(* Logix 5000 AddOnInstructionDefinition export Banner_B25_PD_v4; software revision 33.03 *)

TYPE Banner_B25_PDI_v4 :   // Process Data for a B25. This will include event information.
STRUCT
   Output_State : SINT;   // 0 = Inactive, 1 = Active
   Marginal_Signal : SINT;   // 0 = Normal, 1 = Marginal
END_STRUCT
END_TYPE

ADD_ON_INSTRUCTION Banner_B25_PD_v4   (* revision 4.0, vendor Banner Engineering *)
// Take raw process data and convert it to usable values.
VAR_INPUT
   SINT0 : SINT; {required}
END_VAR
VAR_IN_OUT
   PD : Banner_B25_PDI_v4; {required}
END_VAR

ROUTINE Logic   (* ladder *)
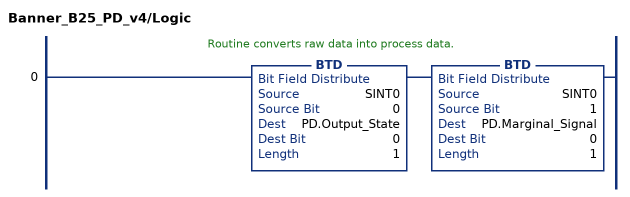
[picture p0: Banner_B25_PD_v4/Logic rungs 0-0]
   // Routine converts raw data into process data.
   0: BTD(SINT0,0,PD.Output_State,0,1)BTD(SINT0,1,PD.Marginal_Signal,0,1);
END_ROUTINE
END_ADD_ON_INSTRUCTION
